(* Logix 5000 AddOnInstructionDefinition export PRNG; software revision 30.00; part 3 of 3 *)
(* tags used below, declared in another part *)
   Out_HASH : LINT[8];
   i : INT;
   HashBuffer_A : LINT;
   HashBuffer_B : LINT;
   HashBuffer_C : LINT;
   HashBuffer_D : LINT;
   HashBuffer_E : LINT;
   HashBuffer_F : LINT;
   HashBuffer_G : LINT;
   HashBuffer_H : LINT;
   HashBufferInput_A : LINT;
   HashBufferInput_B : LINT;
   HashBufferInput_C : LINT;
   HashBufferInput_D : LINT;
   HashBufferInput_E : LINT;
   HashBufferInput_F : LINT;
   HashBufferInput_G : LINT;
   HashBufferInput_H : LINT;
   M : INT;   // MESSAGE INCREMENTS
   t : INT;
   TOTAL_MSG_LENGTH_MINUS_16 : DINT;
(* SHA512_SEQ, continued *)

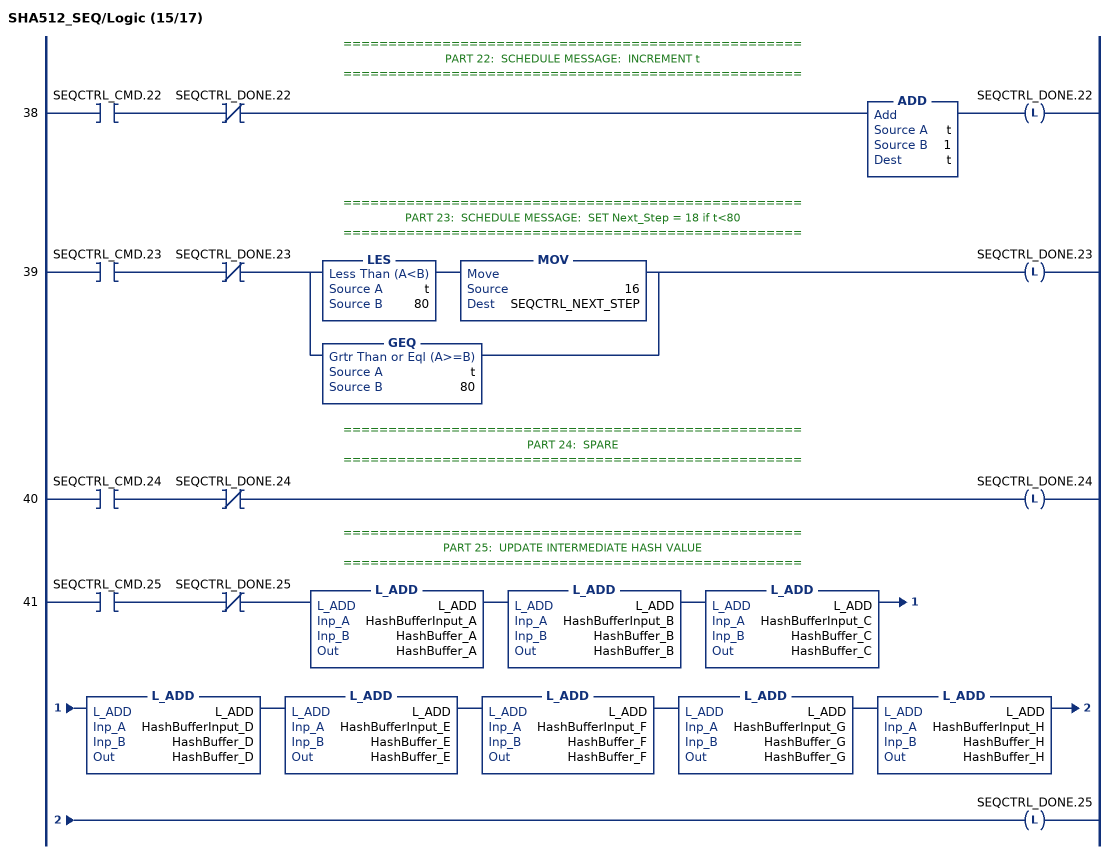
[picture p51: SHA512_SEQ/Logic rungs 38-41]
   // ===================================================
   // PART 22:  SCHEDULE MESSAGE:  INCREMENT t
   // ===================================================
   38: XIC(SEQCTRL_CMD.22)XIO(SEQCTRL_DONE.22)ADD(t,1,t)OTL(SEQCTRL_DONE.22);
   // ===================================================
   // PART 23:  SCHEDULE MESSAGE:  SET Next_Step = 18 if t<80
   // ===================================================
   39: XIC(SEQCTRL_CMD.23)XIO(SEQCTRL_DONE.23)[LES(t,80) MOV(16,SEQCTRL_NEXT_STEP) ,GEQ(t,80) ]OTL(SEQCTRL_DONE.23);
   // ===================================================
   // PART 24:  SPARE
   // ===================================================
   40: XIC(SEQCTRL_CMD.24)XIO(SEQCTRL_DONE.24)OTL(SEQCTRL_DONE.24);
   // ===================================================
   // PART 25:  UPDATE INTERMEDIATE HASH VALUE
   // ===================================================
   41: XIC(SEQCTRL_CMD.25)XIO(SEQCTRL_DONE.25)L_ADD(L_ADD,HashBufferInput_A,HashBuffer_A,HashBuffer_A)L_ADD(L_ADD,HashBufferInput_B,HashBuffer_B,HashBuffer_B)L_ADD(L_ADD,HashBufferInput_C,HashBuffer_C,HashBuffer_C)L_ADD(L_ADD,HashBufferInput_D,HashBuffer_D,HashBuffer_D)L_ADD(L_ADD,HashBufferInput_E,HashBuffer_E,HashBuffer_E)L_ADD(L_ADD,HashBufferInput_F,HashBuffer_F,HashBuffer_F)L_ADD(L_ADD,HashBufferInput_G,HashBuffer_G,HashBuffer_G)L_ADD(L_ADD,HashBufferInput_H,HashBuffer_H,HashBuffer_H)OTL(SEQCTRL_DONE.25);
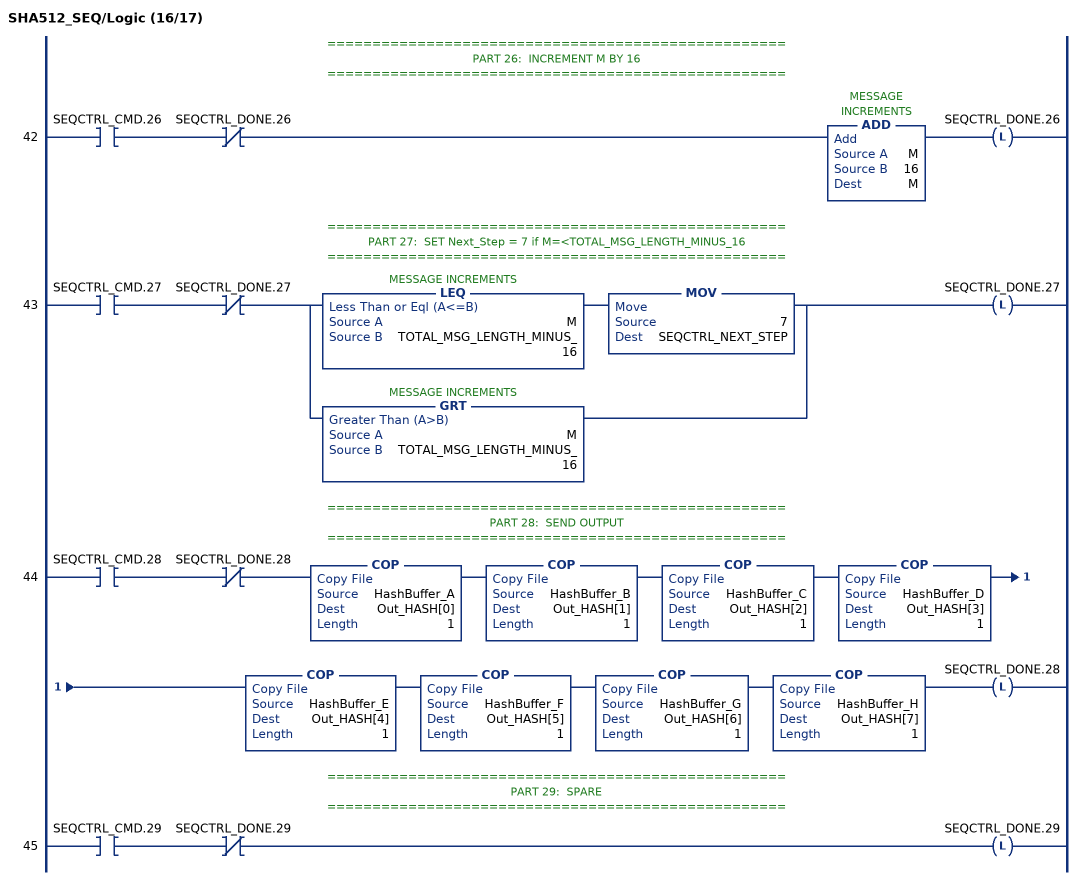
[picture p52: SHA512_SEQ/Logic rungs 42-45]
   // ===================================================
   // PART 26:  INCREMENT M BY 16
   // ===================================================
   42: XIC(SEQCTRL_CMD.26)XIO(SEQCTRL_DONE.26)ADD(M,16,M)OTL(SEQCTRL_DONE.26);
   // ===================================================
   // PART 27:  SET Next_Step = 7 if M=<TOTAL_MSG_LENGTH_MINUS_16
   // ===================================================
   43: XIC(SEQCTRL_CMD.27)XIO(SEQCTRL_DONE.27)[LEQ(M,TOTAL_MSG_LENGTH_MINUS_16) MOV(7,SEQCTRL_NEXT_STEP) ,GRT(M,TOTAL_MSG_LENGTH_MINUS_16) ]OTL(SEQCTRL_DONE.27);
   // ===================================================
   // PART 28:  SEND OUTPUT
   // ===================================================
   44: XIC(SEQCTRL_CMD.28)XIO(SEQCTRL_DONE.28)COP(HashBuffer_A,Out_HASH[0],1)COP(HashBuffer_B,Out_HASH[1],1)COP(HashBuffer_C,Out_HASH[2],1)COP(HashBuffer_D,Out_HASH[3],1)COP(HashBuffer_E,Out_HASH[4],1)COP(HashBuffer_F,Out_HASH[5],1)COP(HashBuffer_G,Out_HASH[6],1)COP(HashBuffer_H,Out_HASH[7],1)OTL(SEQCTRL_DONE.28);
   // ===================================================
   // PART 29:  SPARE
   // ===================================================
   45: XIC(SEQCTRL_CMD.29)XIO(SEQCTRL_DONE.29)OTL(SEQCTRL_DONE.29);
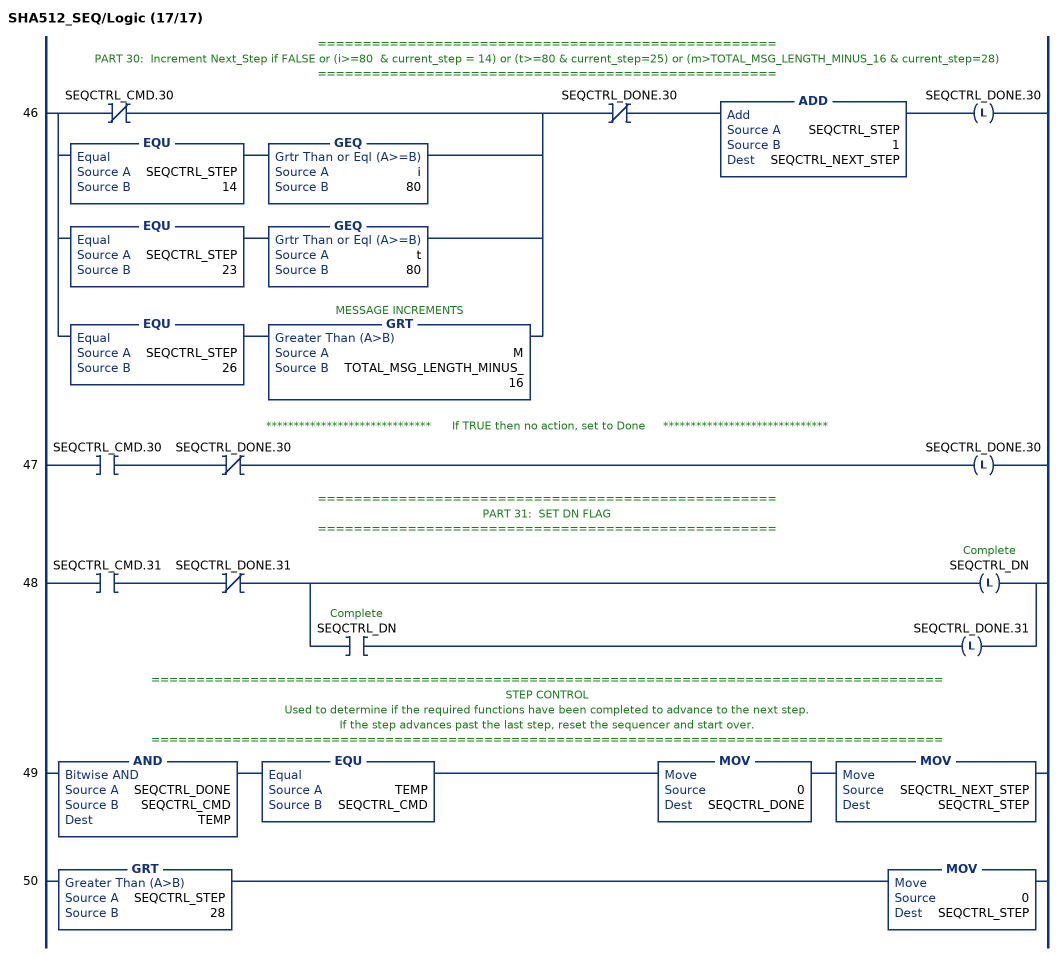
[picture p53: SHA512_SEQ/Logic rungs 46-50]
   // ===================================================
   // PART 30:  Increment Next_Step if FALSE or (i>=80  & current_step = 14) or (t>=80 & current_step=25) or (m>TOTAL_MSG_LENGTH_MINUS_16 & current_step=28)
   // ===================================================
   46: [XIO(SEQCTRL_CMD.30) ,EQU(SEQCTRL_STEP,14) GEQ(i,80) ,EQU(SEQCTRL_STEP,23) GEQ(t,80) ,EQU(SEQCTRL_STEP,26) GRT(M,TOTAL_MSG_LENGTH_MINUS_16) ]XIO(SEQCTRL_DONE.30)ADD(SEQCTRL_STEP,1,SEQCTRL_NEXT_STEP)OTL(SEQCTRL_DONE.30);
   // ******************************      If TRUE then no action, set to Done     ******************************
   47: XIC(SEQCTRL_CMD.30)XIO(SEQCTRL_DONE.30)OTL(SEQCTRL_DONE.30);
   // ===================================================
   // PART 31:  SET DN FLAG
   // ===================================================
   48: XIC(SEQCTRL_CMD.31)XIO(SEQCTRL_DONE.31)[OTL(SEQCTRL_DN) ,XIC(SEQCTRL_DN) OTL(SEQCTRL_DONE.31) ];
   // ========================================================================================
   // STEP CONTROL
   // Used to determine if the required functions have been completed to advance to the next step.
   // If the step advances past the last step, reset the sequencer and start over.
   // ========================================================================================
   49: AND(SEQCTRL_DONE,SEQCTRL_CMD,TEMP)EQU(TEMP,SEQCTRL_CMD)MOV(0,SEQCTRL_DONE)MOV(SEQCTRL_NEXT_STEP,SEQCTRL_STEP);
   50: GRT(SEQCTRL_STEP,28)MOV(0,SEQCTRL_STEP);
END_ROUTINE
END_ADD_ON_INSTRUCTION

ADD_ON_INSTRUCTION L_INC   (* revision 1.0 00 Release, vendor Rockwell Automation *)
// Increment (64-bit)
// Revision note:
// Initial Release
// Help:
// This instruction increments the input 64-bit integer, returning its value plus 1.
VAR_IN_OUT
   Inp : LINT; {required}   // Input
   Out : LINT; {required}   // Output = Input + 1
END_VAR
VAR
   Wrk : DINT[2];   // Working pair of 32-bit integers (DINTs)
   Wrk_LoOvflw : BOOL;   // Low-order 32-bit overflow (without minor fault)
   Wrk_HiOvflw : BOOL;   // High-order 32-bit overflow (without minor fault)
END_VAR

ROUTINE Logic   (* ladder *)
// Output the value of the input plus 1
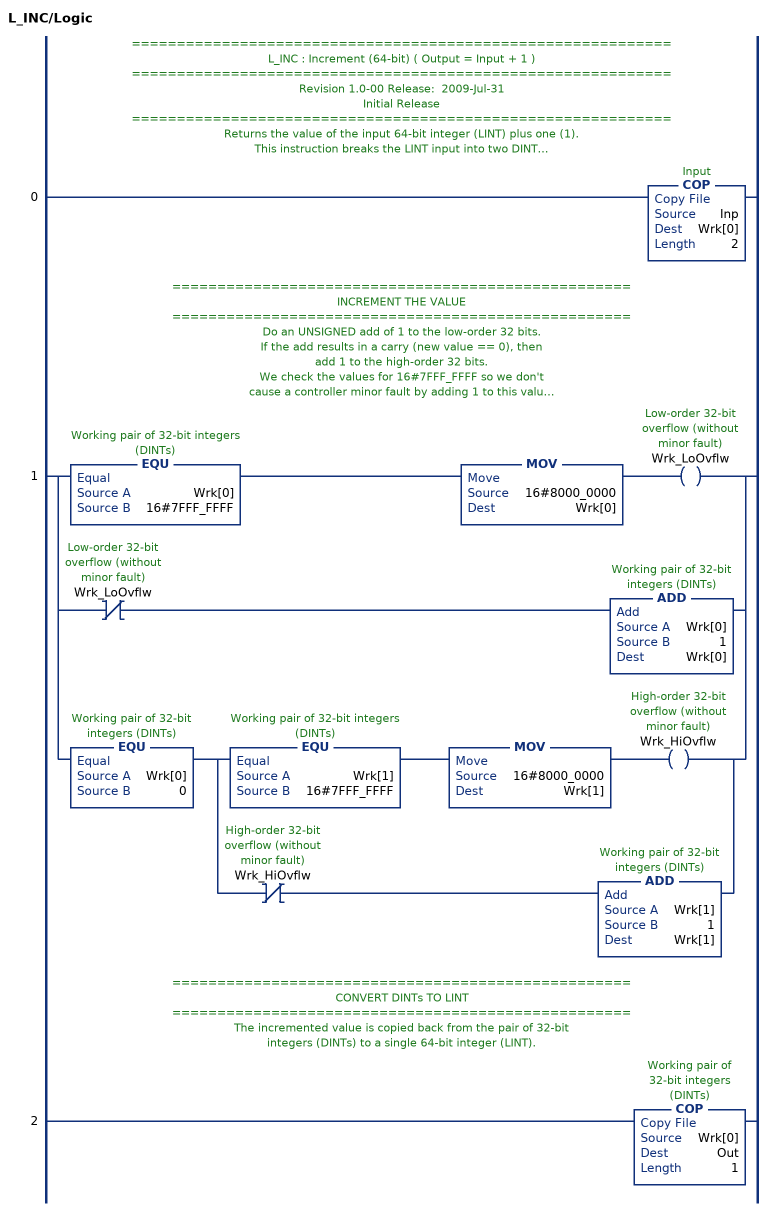
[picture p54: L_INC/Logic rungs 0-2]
   // ============================================================
   // L_INC : Increment (64-bit) ( Output = Input + 1 )
   // ============================================================
   // Revision 1.0-00 Release:  2009-Jul-31
   // Initial Release
   // ============================================================
   // Returns the value of the input 64-bit integer (LINT) plus one (1).
   // This instruction breaks the LINT input into two DINTs
   // (32-bit signed each) to do the math.
   // ===================================================
   // CONVERT LINT TO DINTs
   // ===================================================
   // This COPy takes the input LINT and breaks it into a pair of DINTs.
   0: COP(Inp,Wrk[0],2);
   // ===================================================
   // INCREMENT THE VALUE
   // ===================================================
   // Do an UNSIGNED add of 1 to the low-order 32 bits.
   // If the add results in a carry (new value == 0), then
   // add 1 to the high-order 32 bits.
   // We check the values for 16#7FFF_FFFF so we don't
   // cause a controller minor fault by adding 1 to this value
   // (resulting in a signed overflow to negative).
   1: [EQU(Wrk[0],16#7FFF_FFFF) MOV(16#8000_0000,Wrk[0]) OTE(Wrk_LoOvflw) ,XIO(Wrk_LoOvflw) ADD(Wrk[0],1,Wrk[0]) ,EQU(Wrk[0],0) [EQU(Wrk[1],16#7FFF_FFFF) MOV(16#8000_0000,Wrk[1]) OTE(Wrk_HiOvflw) ,XIO(Wrk_HiOvflw) ADD(Wrk[1],1,Wrk[1]) ] ];
   // ===================================================
   // CONVERT DINTs TO LINT
   // ===================================================
   // The incremented value is copied back from the pair of 32-bit
   // integers (DINTs) to a single 64-bit integer (LINT).
   2: COP(Wrk[0],Out,1);
END_ROUTINE
END_ADD_ON_INSTRUCTION

ADD_ON_INSTRUCTION PRNG   (* revision 1.0 20170916, vendor Kenneth A. Fischer *)
// Pseudo-Random Number Generator
// (not proven secure)
// Revision note:
// Rev1.0: 20170916 - Initial Release
VAR_IN_OUT
   Temp_C : DINT[22]; {required}
   Temp_D : DINT[43]; {required}
   Temp_E : DINT[32]; {required}
   Temp_L : LINT[4]; {required}
   Temp_MSG : LINT[1600]; {required}   // Temp MSG holder
   Temp_HASH : LINT[8]; {required}   // Temp HASH value
   Inp_Constant : STRING; {required}
   Inp_Seed : LINT[13]; {required}
   Inp_Counter : LINT; {required}
   Out_PRN : STRING; {required}
END_VAR
VAR_OUTPUT
   SEQCTRL_DN : BOOL; {access Read Only}   // Complete
END_VAR
VAR_INPUT
   SEQCTRL_RESET : BOOL;   // Resets Ed25519 Verify if Toggled True
END_VAR
VAR_OUTPUT
   SEQCTRL_STEP : INT; {access Read Only}
   SEQCTRL_SUBSTEP : INT; {access Read Only}
END_VAR
VAR
   SEQCTRL_CMD : DINT;
   SEQCTRL_CMD_TABLE : DINT[70];
   SEQCTRL_DONE : DINT;
   SEQCTRL_NEXT_STEP : INT;
   TEMP : DINT;
   SHA512_SEQ : SHA512_SEQ;
   SEQCTRL_ONS : DINT;
   Wrk_Out : DINT[2];
   L_INC : L_INC;
   B256_StoC : B256_StoC;
   B256_CtoE : B256_CtoE;
   B256_EtoL : B256_EtoL;
   B512_HtoD : B512_HtoD;
   B256_CtoS : B256_CtoS;
   L_ROTR : L_ROTR;
   L_ADD : L_ADD;
   SwapLint : LINT;
END_VAR

ROUTINE Logic   (* ladder *)
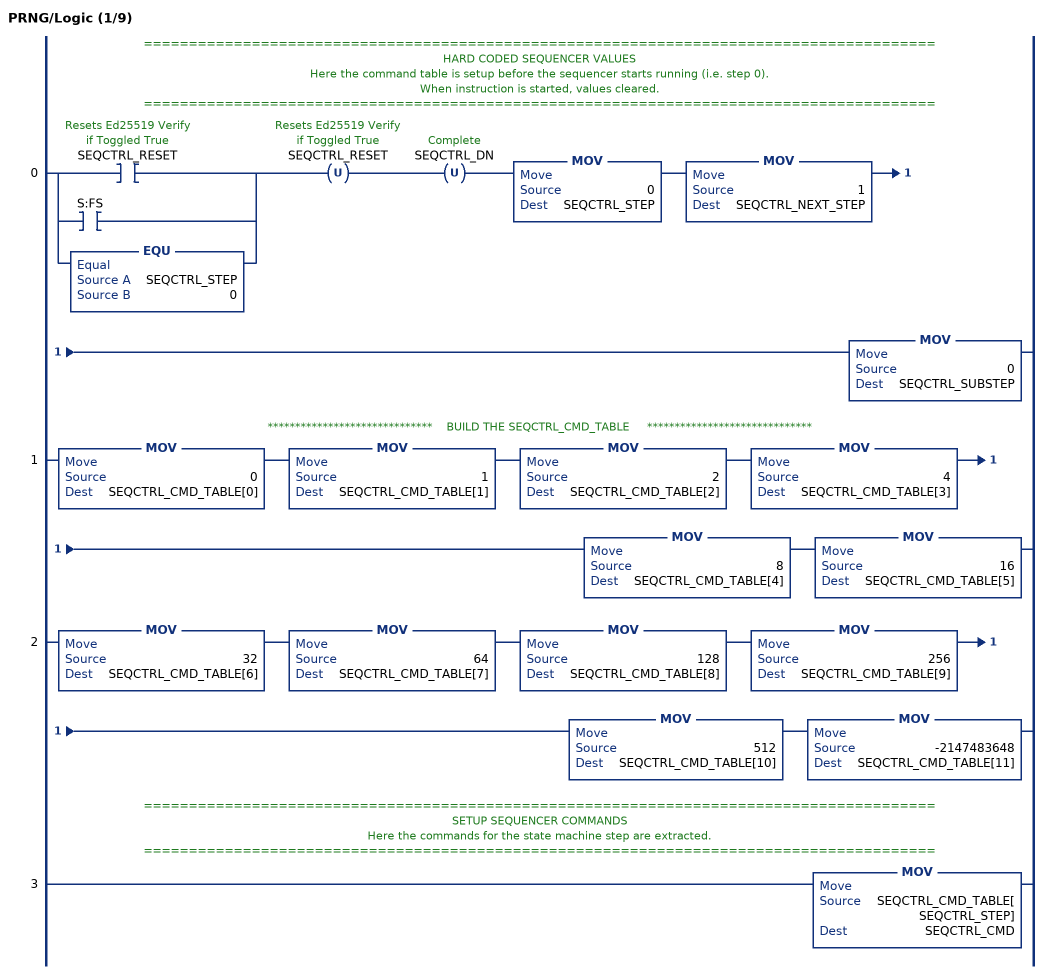
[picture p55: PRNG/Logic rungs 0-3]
   // ========================================================================================
   // HARD CODED SEQUENCER VALUES
   // Here the command table is setup before the sequencer starts running (i.e. step 0).
   // When instruction is started, values cleared.
   // ========================================================================================
   0: [[XIC(SEQCTRL_RESET) ,XIC(S:FS) ] ,EQU(SEQCTRL_STEP,0) ]OTU(SEQCTRL_RESET)OTU(SEQCTRL_DN)MOV(0,SEQCTRL_STEP)MOV(1,SEQCTRL_NEXT_STEP)MOV(0,SEQCTRL_SUBSTEP);
   // ******************************    BUILD THE SEQCTRL_CMD_TABLE     ******************************
   1: MOV(0,SEQCTRL_CMD_TABLE[0])MOV(1,SEQCTRL_CMD_TABLE[1])MOV(2,SEQCTRL_CMD_TABLE[2])MOV(4,SEQCTRL_CMD_TABLE[3])MOV(8,SEQCTRL_CMD_TABLE[4])MOV(16,SEQCTRL_CMD_TABLE[5]);
   2: MOV(32,SEQCTRL_CMD_TABLE[6])MOV(64,SEQCTRL_CMD_TABLE[7])MOV(128,SEQCTRL_CMD_TABLE[8])MOV(256,SEQCTRL_CMD_TABLE[9])MOV(512,SEQCTRL_CMD_TABLE[10])MOV(-2147483648,SEQCTRL_CMD_TABLE[11]);
   // ========================================================================================
   // SETUP SEQUENCER COMMANDS
   // Here the commands for the state machine step are extracted.
   // ========================================================================================
   3: MOV(SEQCTRL_CMD_TABLE[SEQCTRL_STEP],SEQCTRL_CMD);
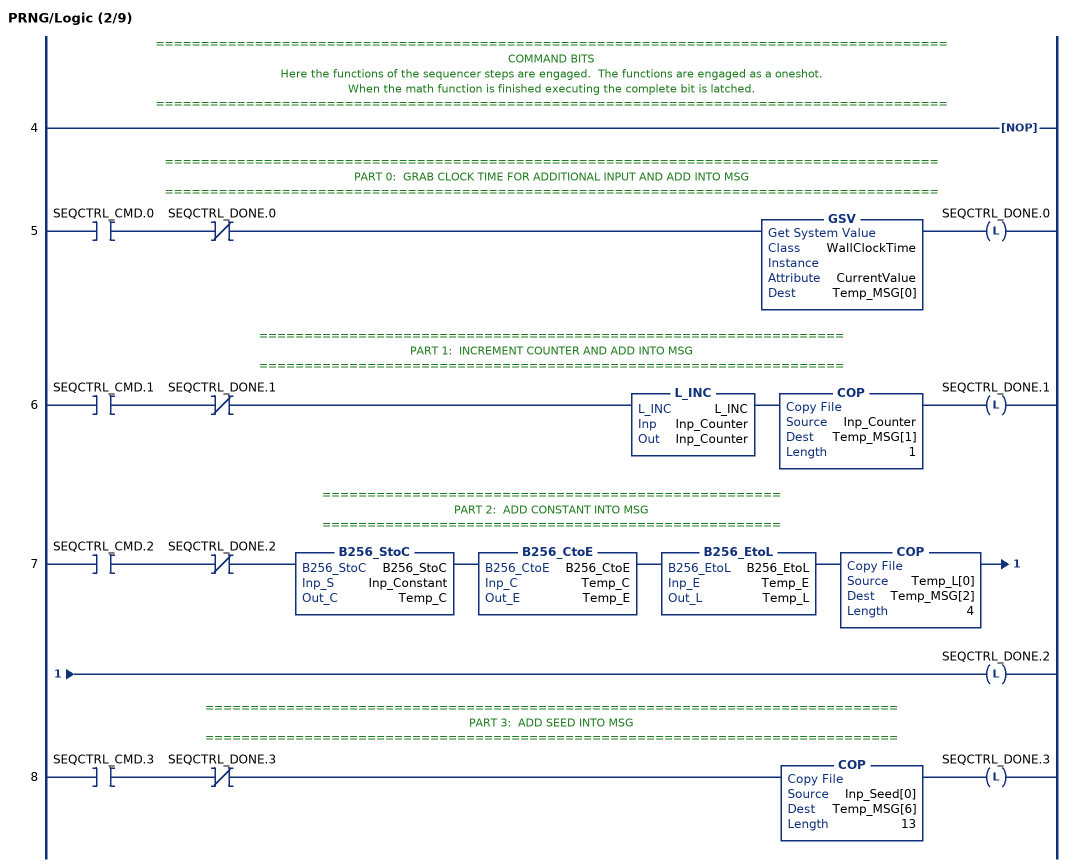
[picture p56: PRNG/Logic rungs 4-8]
   // ========================================================================================
   // COMMAND BITS
   // Here the functions of the sequencer steps are engaged.  The functions are engaged as a oneshot.
   // When the math function is finished executing the complete bit is latched.
   // ========================================================================================
   4: NOP();
   // ======================================================================================
   // PART 0:  GRAB CLOCK TIME FOR ADDITIONAL INPUT AND ADD INTO MSG
   // ======================================================================================
   5: XIC(SEQCTRL_CMD.0)XIO(SEQCTRL_DONE.0)GSV(WallClockTime,,CurrentValue,Temp_MSG[0])OTL(SEQCTRL_DONE.0);
   // =================================================================
   // PART 1:  INCREMENT COUNTER AND ADD INTO MSG
   // =================================================================
   6: XIC(SEQCTRL_CMD.1)XIO(SEQCTRL_DONE.1)L_INC(L_INC,Inp_Counter,Inp_Counter)COP(Inp_Counter,Temp_MSG[1],1)OTL(SEQCTRL_DONE.1);
   // ===================================================
   // PART 2:  ADD CONSTANT INTO MSG
   // ===================================================
   7: XIC(SEQCTRL_CMD.2)XIO(SEQCTRL_DONE.2)B256_StoC(B256_StoC,Inp_Constant,Temp_C)B256_CtoE(B256_CtoE,Temp_C,Temp_E)B256_EtoL(B256_EtoL,Temp_E,Temp_L)COP(Temp_L[0],Temp_MSG[2],4)OTL(SEQCTRL_DONE.2);
   // =============================================================================
   // PART 3:  ADD SEED INTO MSG
   // =============================================================================
   8: XIC(SEQCTRL_CMD.3)XIO(SEQCTRL_DONE.3)COP(Inp_Seed[0],Temp_MSG[6],13)OTL(SEQCTRL_DONE.3);
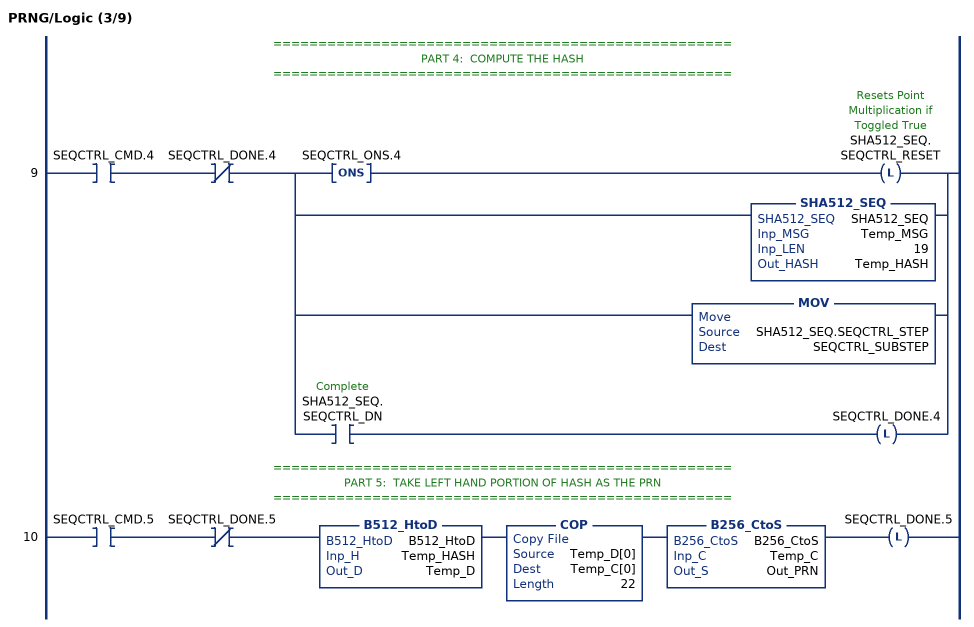
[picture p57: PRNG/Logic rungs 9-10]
   // ===================================================
   // PART 4:  COMPUTE THE HASH
   // ===================================================
   9: XIC(SEQCTRL_CMD.4)XIO(SEQCTRL_DONE.4)[ONS(SEQCTRL_ONS.4) OTL(SHA512_SEQ.SEQCTRL_RESET) ,SHA512_SEQ(SHA512_SEQ,Temp_MSG,19,Temp_HASH) ,MOV(SHA512_SEQ.SEQCTRL_STEP,SEQCTRL_SUBSTEP) ,XIC(SHA512_SEQ.SEQCTRL_DN) OTL(SEQCTRL_DONE.4) ];
   // ===================================================
   // PART 5:  TAKE LEFT HAND PORTION OF HASH AS THE PRN
   // ===================================================
   10: XIC(SEQCTRL_CMD.5)XIO(SEQCTRL_DONE.5)B512_HtoD(B512_HtoD,Temp_HASH,Temp_D)COP(Temp_D[0],Temp_C[0],22)B256_CtoS(B256_CtoS,Temp_C,Out_PRN)OTL(SEQCTRL_DONE.5);
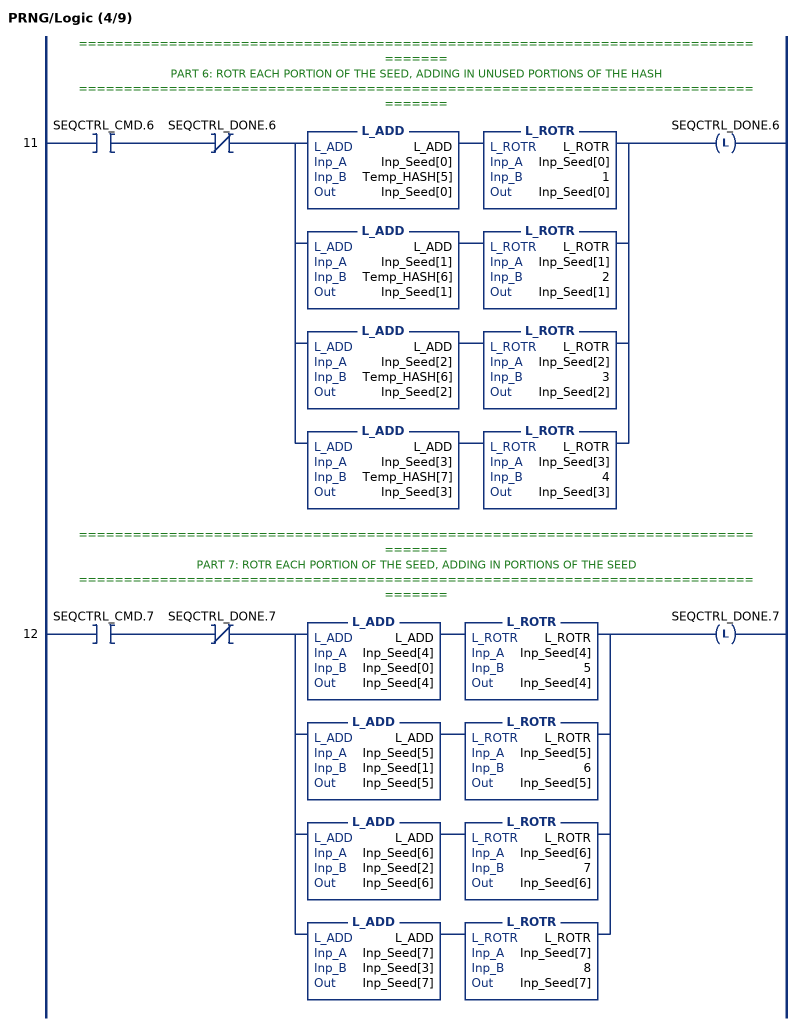
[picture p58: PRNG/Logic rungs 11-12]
   // ==================================================================================
   // PART 6: ROTR EACH PORTION OF THE SEED, ADDING IN UNUSED PORTIONS OF THE HASH
   // ==================================================================================
   11: XIC(SEQCTRL_CMD.6)XIO(SEQCTRL_DONE.6)[L_ADD(L_ADD,Inp_Seed[0],Temp_HASH[5],Inp_Seed[0]) L_ROTR(L_ROTR,Inp_Seed[0],1,Inp_Seed[0]) ,L_ADD(L_ADD,Inp_Seed[1],Temp_HASH[6],Inp_Seed[1]) L_ROTR(L_ROTR,Inp_Seed[1],2,Inp_Seed[1]) ,L_ADD(L_ADD,Inp_Seed[2],Temp_HASH[6],Inp_Seed[2]) L_ROTR(L_ROTR,Inp_Seed[2],3,Inp_Seed[2]) ,L_ADD(L_ADD,Inp_Seed[3],Temp_HASH[7],Inp_Seed[3]) L_ROTR(L_ROTR,Inp_Seed[3],4,Inp_Seed[3]) ]OTL(SEQCTRL_DONE.6);
   // ==================================================================================
   // PART 7: ROTR EACH PORTION OF THE SEED, ADDING IN PORTIONS OF THE SEED
   // ==================================================================================
   12: XIC(SEQCTRL_CMD.7)XIO(SEQCTRL_DONE.7)[L_ADD(L_ADD,Inp_Seed[4],Inp_Seed[0],Inp_Seed[4]) L_ROTR(L_ROTR,Inp_Seed[4],5,Inp_Seed[4]) ,L_ADD(L_ADD,Inp_Seed[5],Inp_Seed[1],Inp_Seed[5]) L_ROTR(L_ROTR,Inp_Seed[5],6,Inp_Seed[5]) ,L_ADD(L_ADD,Inp_Seed[6],Inp_Seed[2],Inp_Seed[6]) L_ROTR(L_ROTR,Inp_Seed[6],7,Inp_Seed[6]) ,L_ADD(L_ADD,Inp_Seed[7],Inp_Seed[3],Inp_Seed[7]) L_ROTR(L_ROTR,Inp_Seed[7],8,Inp_Seed[7]) ]OTL(SEQCTRL_DONE.7);
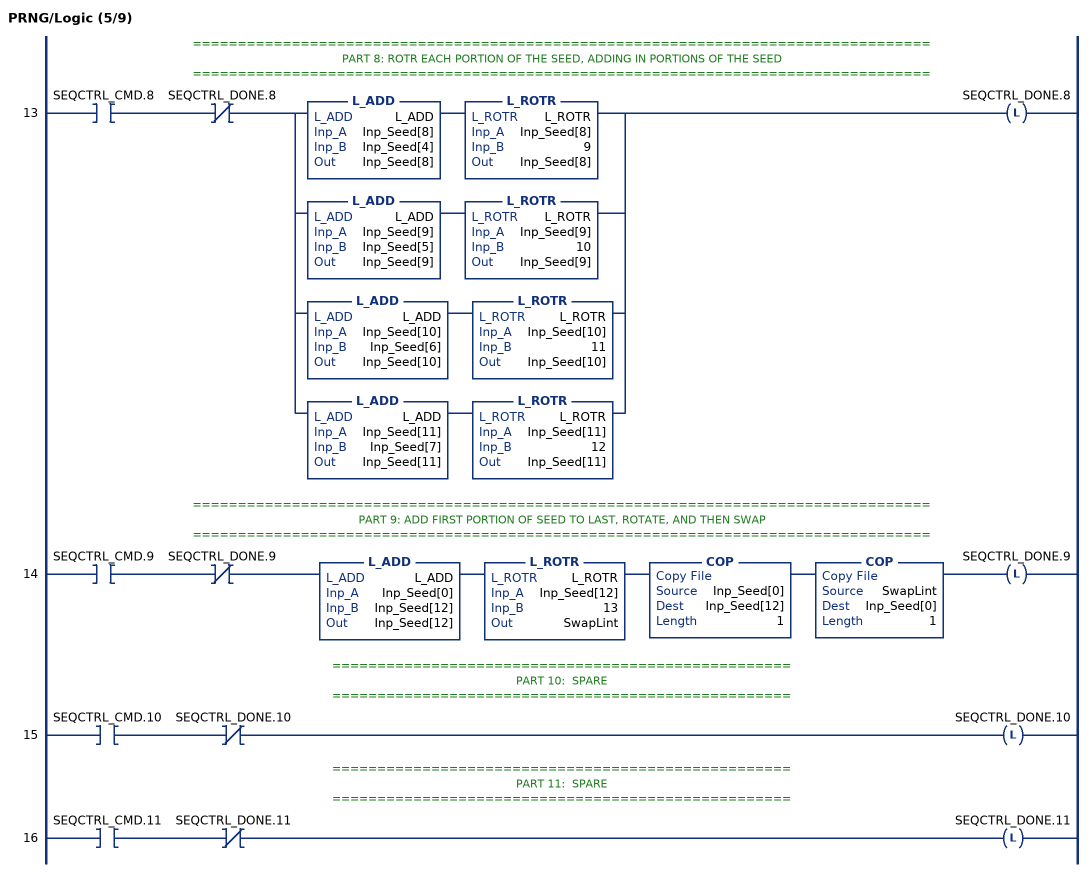
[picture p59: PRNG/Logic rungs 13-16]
   // ==================================================================================
   // PART 8: ROTR EACH PORTION OF THE SEED, ADDING IN PORTIONS OF THE SEED
   // ==================================================================================
   13: XIC(SEQCTRL_CMD.8)XIO(SEQCTRL_DONE.8)[L_ADD(L_ADD,Inp_Seed[8],Inp_Seed[4],Inp_Seed[8]) L_ROTR(L_ROTR,Inp_Seed[8],9,Inp_Seed[8]) ,L_ADD(L_ADD,Inp_Seed[9],Inp_Seed[5],Inp_Seed[9]) L_ROTR(L_ROTR,Inp_Seed[9],10,Inp_Seed[9]) ,L_ADD(L_ADD,Inp_Seed[10],Inp_Seed[6],Inp_Seed[10]) L_ROTR(L_ROTR,Inp_Seed[10],11,Inp_Seed[10]) ,L_ADD(L_ADD,Inp_Seed[11],Inp_Seed[7],Inp_Seed[11]) L_ROTR(L_ROTR,Inp_Seed[11],12,Inp_Seed[11]) ]OTL(SEQCTRL_DONE.8);
   // ==================================================================================
   // PART 9: ADD FIRST PORTION OF SEED TO LAST, ROTATE, AND THEN SWAP
   // ==================================================================================
   14: XIC(SEQCTRL_CMD.9)XIO(SEQCTRL_DONE.9)L_ADD(L_ADD,Inp_Seed[0],Inp_Seed[12],Inp_Seed[12])L_ROTR(L_ROTR,Inp_Seed[12],13,SwapLint)COP(Inp_Seed[0],Inp_Seed[12],1)COP(SwapLint,Inp_Seed[0],1)OTL(SEQCTRL_DONE.9);
   // ===================================================
   // PART 10:  SPARE
   // ===================================================
   15: XIC(SEQCTRL_CMD.10)XIO(SEQCTRL_DONE.10)OTL(SEQCTRL_DONE.10);
   // ===================================================
   // PART 11:  SPARE
   // ===================================================
   16: XIC(SEQCTRL_CMD.11)XIO(SEQCTRL_DONE.11)OTL(SEQCTRL_DONE.11);
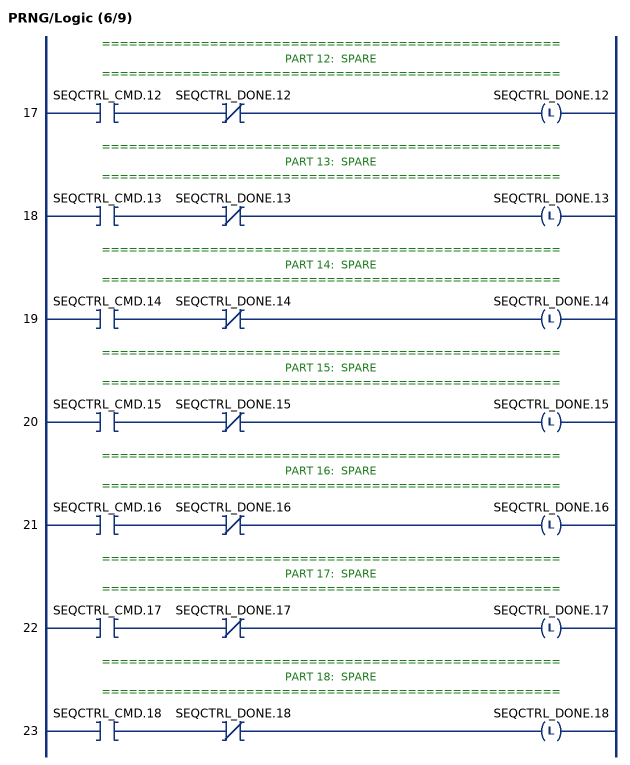
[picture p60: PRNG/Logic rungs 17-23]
   // ===================================================
   // PART 12:  SPARE
   // ===================================================
   17: XIC(SEQCTRL_CMD.12)XIO(SEQCTRL_DONE.12)OTL(SEQCTRL_DONE.12);
   // ===================================================
   // PART 13:  SPARE
   // ===================================================
   18: XIC(SEQCTRL_CMD.13)XIO(SEQCTRL_DONE.13)OTL(SEQCTRL_DONE.13);
   // ===================================================
   // PART 14:  SPARE
   // ===================================================
   19: XIC(SEQCTRL_CMD.14)XIO(SEQCTRL_DONE.14)OTL(SEQCTRL_DONE.14);
   // ===================================================
   // PART 15:  SPARE
   // ===================================================
   20: XIC(SEQCTRL_CMD.15)XIO(SEQCTRL_DONE.15)OTL(SEQCTRL_DONE.15);
   // ===================================================
   // PART 16:  SPARE
   // ===================================================
   21: XIC(SEQCTRL_CMD.16)XIO(SEQCTRL_DONE.16)OTL(SEQCTRL_DONE.16);
   // ===================================================
   // PART 17:  SPARE
   // ===================================================
   22: XIC(SEQCTRL_CMD.17)XIO(SEQCTRL_DONE.17)OTL(SEQCTRL_DONE.17);
   // ===================================================
   // PART 18:  SPARE
   // ===================================================
   23: XIC(SEQCTRL_CMD.18)XIO(SEQCTRL_DONE.18)OTL(SEQCTRL_DONE.18);
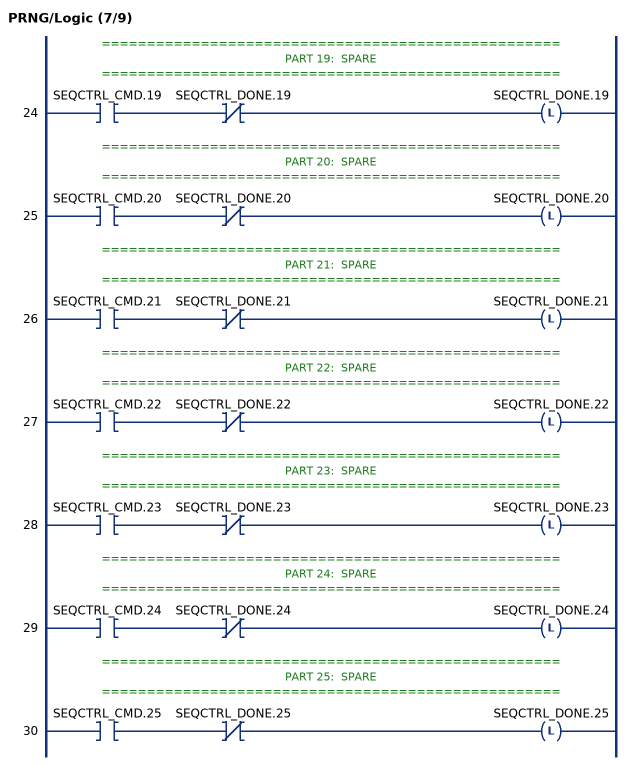
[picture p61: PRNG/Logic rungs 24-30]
   // ===================================================
   // PART 19:  SPARE
   // ===================================================
   24: XIC(SEQCTRL_CMD.19)XIO(SEQCTRL_DONE.19)OTL(SEQCTRL_DONE.19);
   // ===================================================
   // PART 20:  SPARE
   // ===================================================
   25: XIC(SEQCTRL_CMD.20)XIO(SEQCTRL_DONE.20)OTL(SEQCTRL_DONE.20);
   // ===================================================
   // PART 21:  SPARE
   // ===================================================
   26: XIC(SEQCTRL_CMD.21)XIO(SEQCTRL_DONE.21)OTL(SEQCTRL_DONE.21);
   // ===================================================
   // PART 22:  SPARE
   // ===================================================
   27: XIC(SEQCTRL_CMD.22)XIO(SEQCTRL_DONE.22)OTL(SEQCTRL_DONE.22);
   // ===================================================
   // PART 23:  SPARE
   // ===================================================
   28: XIC(SEQCTRL_CMD.23)XIO(SEQCTRL_DONE.23)OTL(SEQCTRL_DONE.23);
   // ===================================================
   // PART 24:  SPARE
   // ===================================================
   29: XIC(SEQCTRL_CMD.24)XIO(SEQCTRL_DONE.24)OTL(SEQCTRL_DONE.24);
   // ===================================================
   // PART 25:  SPARE
   // ===================================================
   30: XIC(SEQCTRL_CMD.25)XIO(SEQCTRL_DONE.25)OTL(SEQCTRL_DONE.25);
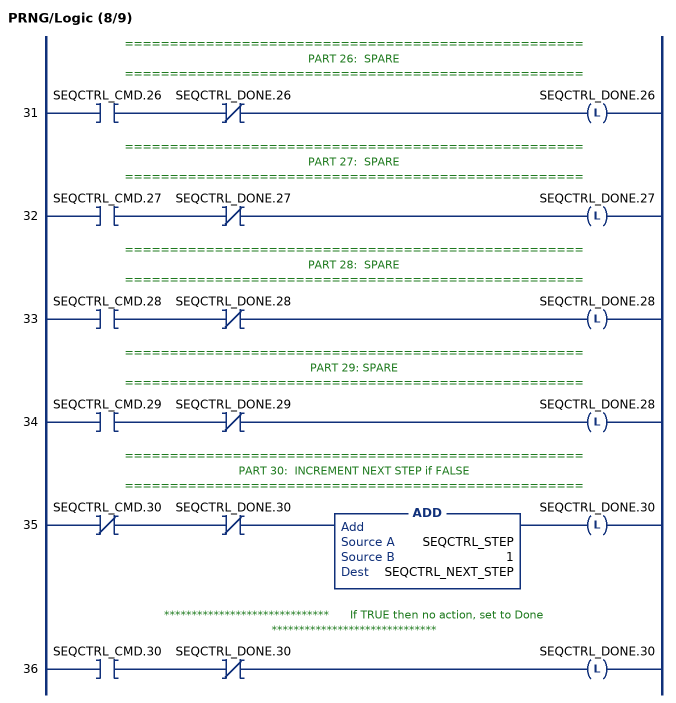
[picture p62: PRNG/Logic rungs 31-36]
   // ===================================================
   // PART 26:  SPARE
   // ===================================================
   31: XIC(SEQCTRL_CMD.26)XIO(SEQCTRL_DONE.26)OTL(SEQCTRL_DONE.26);
   // ===================================================
   // PART 27:  SPARE
   // ===================================================
   32: XIC(SEQCTRL_CMD.27)XIO(SEQCTRL_DONE.27)OTL(SEQCTRL_DONE.27);
   // ===================================================
   // PART 28:  SPARE
   // ===================================================
   33: XIC(SEQCTRL_CMD.28)XIO(SEQCTRL_DONE.28)OTL(SEQCTRL_DONE.28);
   // ===================================================
   // PART 29: SPARE
   // ===================================================
   34: XIC(SEQCTRL_CMD.29)XIO(SEQCTRL_DONE.29)OTL(SEQCTRL_DONE.28);
   // ===================================================
   // PART 30:  INCREMENT NEXT STEP if FALSE
   // ===================================================
   35: XIO(SEQCTRL_CMD.30)XIO(SEQCTRL_DONE.30)ADD(SEQCTRL_STEP,1,SEQCTRL_NEXT_STEP)OTL(SEQCTRL_DONE.30);
   // ******************************      If TRUE then no action, set to Done     ******************************
   36: XIC(SEQCTRL_CMD.30)XIO(SEQCTRL_DONE.30)OTL(SEQCTRL_DONE.30);
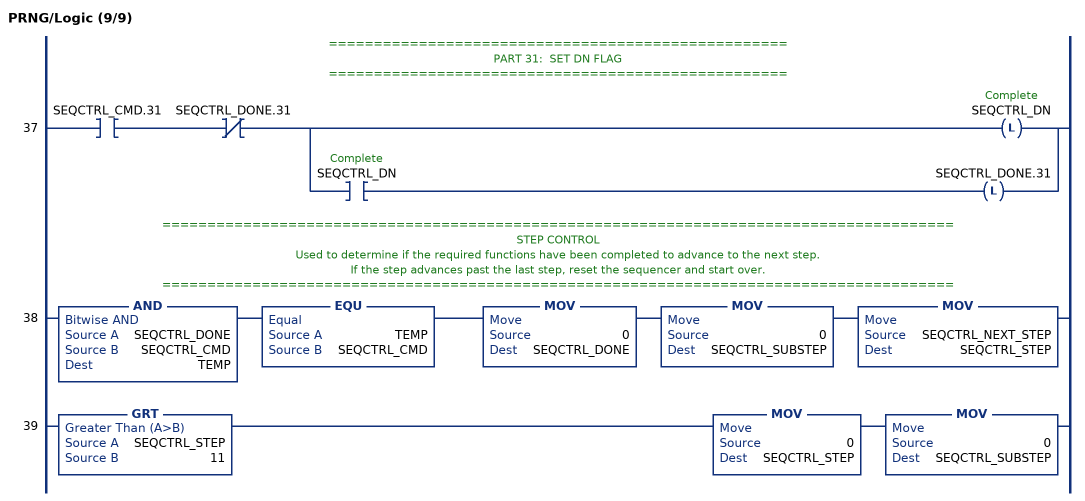
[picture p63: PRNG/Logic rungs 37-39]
   // ===================================================
   // PART 31:  SET DN FLAG
   // ===================================================
   37: XIC(SEQCTRL_CMD.31)XIO(SEQCTRL_DONE.31)[OTL(SEQCTRL_DN) ,XIC(SEQCTRL_DN) OTL(SEQCTRL_DONE.31) ];
   // ========================================================================================
   // STEP CONTROL
   // Used to determine if the required functions have been completed to advance to the next step.
   // If the step advances past the last step, reset the sequencer and start over.
   // ========================================================================================
   38: AND(SEQCTRL_DONE,SEQCTRL_CMD,TEMP)EQU(TEMP,SEQCTRL_CMD)MOV(0,SEQCTRL_DONE)MOV(0,SEQCTRL_SUBSTEP)MOV(SEQCTRL_NEXT_STEP,SEQCTRL_STEP);
   39: GRT(SEQCTRL_STEP,11)MOV(0,SEQCTRL_STEP)MOV(0,SEQCTRL_SUBSTEP);
END_ROUTINE
END_ADD_ON_INSTRUCTION
